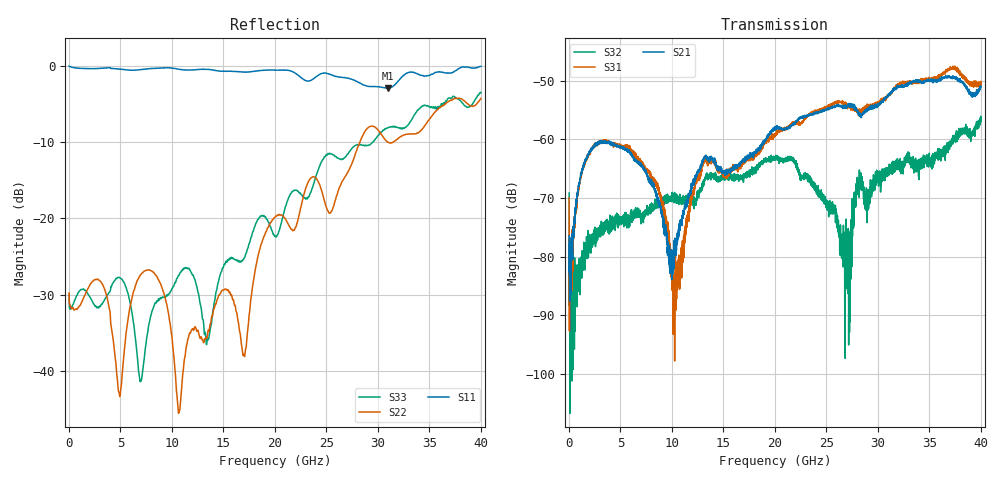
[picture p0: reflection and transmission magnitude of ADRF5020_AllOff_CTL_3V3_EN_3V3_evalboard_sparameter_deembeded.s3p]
! Device:  ADRF5020
! Description: SOI MMIC SPDT Non-Reflective Switch
! Frequency:  0.1 -  30 GHz
! Ports:
! 	RFC	= Port 1
!	RF1	= Port 2
!	RF2	= Port 3
! Vdd:  +3.3 Volt
! Vss:  -2.5 Volt
! Control:  0/+3.3 Volt
! State:  All Off (Vctl= 3.3 V, Ven= 3.3 V)
! Data:	Data was collected using a calibrated network analyzer with AFR software.
!	Fixtures were calculated using AFR and fixturing was applied to collect
!	this Deembedded  S Parameter data of ADRF5020.
! Note:	Analog Devices supplies this data as a sample of measured data at the package pin
!	for this product.  Your particular data for this product may vary.
!	Data was taken at 25 degrees C.
!	Analog Devices reserves the right to change this data at anytime.
# Hz S  dB  R 50
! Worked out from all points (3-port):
!   4000 points, 10 MHz to 40 GHz, reference 50 ohm
!   strongest paths, dB at 10 MHz, 10.01 GHz, 20.01 GHz, 30.01 GHz, 40 GHz:
!     S21: -76.5, -81.5, -58.2, -54.2, -51.0
!     S31: -70.0, -83.1, -59.1, -53.6, -50.7
!     S32: -69.2, -69.4, -63.6, -65.8, -57.0
!   lowest |S11| = -3.0 dB at 31 GHz (marker M1), VSWR 5.92, Z = 77.5 - j123 ohm
!   |S11| at or under -10 dB: nowhere
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1e7  -0.08 -0.4  -72.42 -67.3  -75.02 29.3
     -76.48 106.1  -29.73 148.0  -86.94 99.1
     -70.00 -29.1  -69.16 -95.5  -30.04 146.8
2.98e9  -0.37 -36.8  -60.53 39.4  -60.67 38.9
        -60.48 40.1  -28.12 168.8  -74.81 74.4
        -60.64 39.6  -75.45 72.5  -31.48 168.1
4.91e9  -0.47 -54.2  -61.05 24.9  -61.08 20.9
        -61.36 23.9  -43.16 161.6  -73.95 75.1
        -60.77 21.4  -73.51 72.4  -27.70 -152.7
6.94e9  -0.53 -79.6  -64.38 10.4  -63.84 4.3
        -63.99 11.0  -27.35 155.2  -73.05 77.1
        -63.79 2.3  -73.39 83.0  -41.24 -138.8
9.15e9  -0.31 -103.4  -73.76 5.6  -71.92 -6.8
        -74.23 12.4  -29.55 -127.0  -70.09 88.2
        -72.34 -13.2  -70.75 84.6  -30.29 -143.5
1.07e10  -0.49 -116.8  -74.97 119.6  -82.96 108.1
         -74.38 121.5  -45.25 25.6  -70.24 79.8
         -80.66 116.5  -70.56 79.2  -27.39 -119.7
2.001e10  -0.60 146.7  -58.26 123.1  -59.33 116.0
          -58.23 123.2  -19.82 -29.5  -62.98 -18.9
          -59.11 116.0  -63.58 -20.8  -22.32 -42.7
2.519e10  -1.08 71.3  -54.59 101.1  -54.38 95.0
          -54.58 101.3  -19.13 -34.4  -72.44 -87.9
          -54.43 94.5  -71.65 -80.5  -11.53 -66.1
3.1e10  -2.96 -33.4  -52.50 61.4  -52.61 55.7
        -52.50 62.2  -10.02 -66.2  -64.73 -74.5
        -52.48 56.8  -65.02 -74.6  -8.11 -92.8
4e10  -0.10 -137.5  -51.05 6.7  -50.59 -9.8
      -51.04 6.2  -4.30 -118.4  -57.15 118.1
      -50.74 -10.5  -57.01 117.5  -3.51 -137.6
